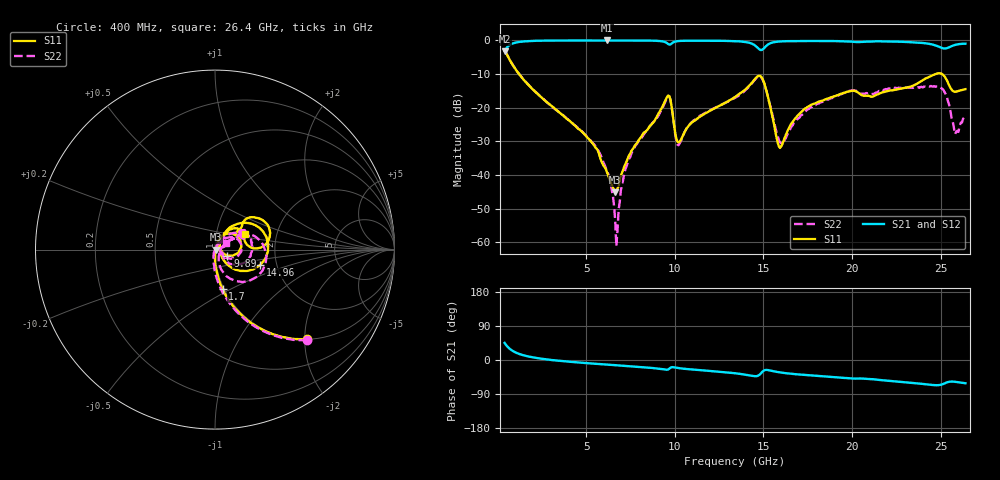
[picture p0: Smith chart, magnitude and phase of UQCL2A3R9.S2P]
! AVX Corporation
! Date:  10/27/06
! Part No:  UQCL2A3R9
! Description:  Ultra Low ESR Microwave capacitors
! Mounting Orientation:  Horizontal
# GHZ S DB R 50
! Freq  |S11|  S11 Ph  |S21|  S21 Ph  |S12|  S12 Ph  |S22|  S22 Ph
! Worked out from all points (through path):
!   401 points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, 400 MHz to 26.4 GHz, reference 50 ohm
!   highest |S21| = -0.03 dB at 6.185 GHz (marker M1); lowest = -3.2 dB at 400 MHz (marker M2)
!   group delay of S21, straight-line fit = 8.17 ps
!   lowest |S11| = -45.1 dB at 6.64 GHz (marker M3), VSWR 1.01, Z = 50.6 - j0.0775 ohm
!   |S11| at or under -10 dB: 1.212 GHz to 24.73 GHz (23.51 GHz wide, 181 % of centre); 25.08 GHz to end of sweep
!   |S22| runs from -61.2 to -2.8 dB; largest |S21 - S12| = 0.0086
!   S11 on the Smith chart (normalised r, x): 400 MHz: 1.00, -2.05; 1.7 GHz: 0.98, -0.46; 9.89 GHz: 1.15, -0.08; 14.96 GHz: 1.63, -0.30; 26.4 GHz: 1.37, +0.25
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0.4  -2.91 -44.4  -3.22 45.0  -3.19 45.0  -2.84 -44.6
1.7  -13.00 -79.2  -0.23 9.7  -0.20 9.6  -12.95 -81.2
4.755  -27.11 -90.0  -0.04 -7.3  -0.02 -7.5  -26.97 -101.2
6.185  -39.34 -66.1  -0.03 -12.2  -0.04 -12.4  -38.96 -109.6
6.64  -45.12 -7.9  -0.04 -13.7  -0.04 -14.0  -53.36 -126.5
6.77  -44.03 20.2  -0.04 -14.1  -0.05 -14.4  -56.36 76.3
7.095  -38.37 50.7  -0.04 -15.2  -0.05 -15.5  -41.25 69.0
7.485  -33.62 61.5  -0.04 -16.5  -0.06 -16.9  -34.70 64.6
9.11  -21.48 64.1  -0.17 -23.1  -0.21 -23.4  -22.10 48.7
9.63  -16.42 20.8  -1.09 -24.9  -1.13 -25.3  -16.53 11.3
9.89  -22.27 -25.5  -0.68 -18.8  -0.71 -19.2  -22.22 -36.5
10.215  -30.34 19.7  -0.20 -21.3  -0.24 -21.6  -31.16 11.5
11.125  -23.88 57.2  -0.10 -25.6  -0.12 -25.7  -23.63 52.8
13.4  -16.83 56.6  -0.23 -34.9  -0.26 -35.0  -17.09 41.2
14.44  -12.03 35.1  -1.21 -42.3  -1.25 -42.4  -12.22 14.9
14.96  -11.52 -19.0  -2.72 -30.2  -2.75 -30.2  -11.68 -41.0
15.935  -31.96 4.3  -0.33 -32.7  -0.36 -32.7  -30.31 -35.2
17.755  -19.03 58.6  -0.19 -40.9  -0.24 -40.8  -19.79 31.6
22.11  -14.93 39.1  -0.36 -54.9  -0.40 -54.5  -14.25 35.3
24.905  -9.77 23.1  -1.90 -66.3  -1.93 -65.8  -13.93 -6.1
25.88  -15.24 19.0  -1.27 -57.9  -1.30 -57.5  -27.18 -9.2
26.4  -14.51 28.1  -0.99 -61.3  -1.01 -60.9  -23.03 28.8
